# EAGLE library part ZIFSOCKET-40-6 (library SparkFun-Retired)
Lever-action ZIF socket for 40-pin ICs
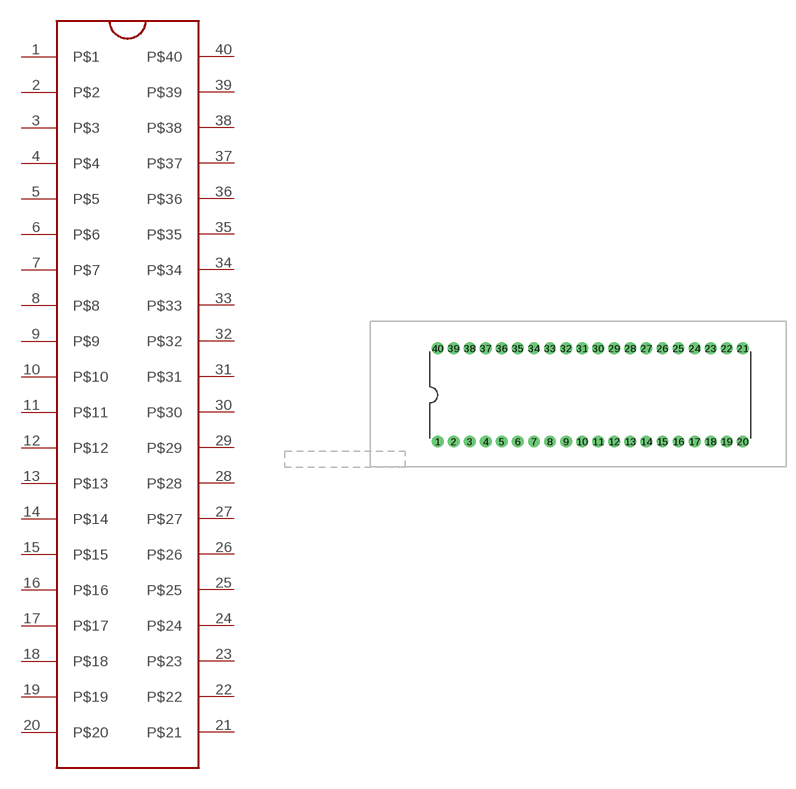
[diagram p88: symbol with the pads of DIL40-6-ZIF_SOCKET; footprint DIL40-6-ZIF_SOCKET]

Designator prefix -

## ZIFSOCKET-40-6DIL40-6-ZIF_SOCKET  [DIL40-6-ZIF_SOCKET]
1  P$1
2  P$2
3  P$3
4  P$4
5  P$5
6  P$6
7  P$7
8  P$8
9  P$9
10  P$10
11  P$11
12  P$12
13  P$13
14  P$14
15  P$15
16  P$16
17  P$17
18  P$18
19  P$19
20  P$20
21  P$21
22  P$22
23  P$23
24  P$24
25  P$25
26  P$26
27  P$27
28  P$28
29  P$29
30  P$30
31  P$31
32  P$32
33  P$33
34  P$34
35  P$35
36  P$36
37  P$37
38  P$38
39  P$39
40  P$40

## Footprint DIL40-6-ZIF_SOCKET (pad centres in mm)
drill 1.016 pad 1.88: 1 -24.13,-7.366; 2 -21.59,-7.366; 3 -19.05,-7.366; 4 -16.51,-7.366; 5 -13.97,-7.366; 6 -11.43,-7.366; 7 -8.89,-7.366; 8 -6.35,-7.366; 9 -3.81,-7.366; 10 -1.27,-7.366; 11 1.27,-7.366; 12 3.81,-7.366; 13 6.35,-7.366; 14 8.89,-7.366; 15 11.43,-7.366; 16 13.97,-7.366; 17 16.51,-7.366; 18 19.05,-7.366; 19 21.59,-7.366; 20 24.13,-7.366; 21 24.13,7.366; 22 21.59,7.366; 23 19.05,7.366; 24 16.51,7.366; 25 13.97,7.366; 26 11.43,7.366; 27 8.89,7.366; 28 6.35,7.366
drill 1.1 pad 1.88: 29 3.81,7.366; 30 1.27,7.366; 31 -1.27,7.366; 32 -3.81,7.366; 33 -6.35,7.366; 34 -8.89,7.366; 35 -11.43,7.366; 36 -13.97,7.366; 37 -16.51,7.366; 38 -19.05,7.366; 39 -21.59,7.366; 40 -24.13,7.366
